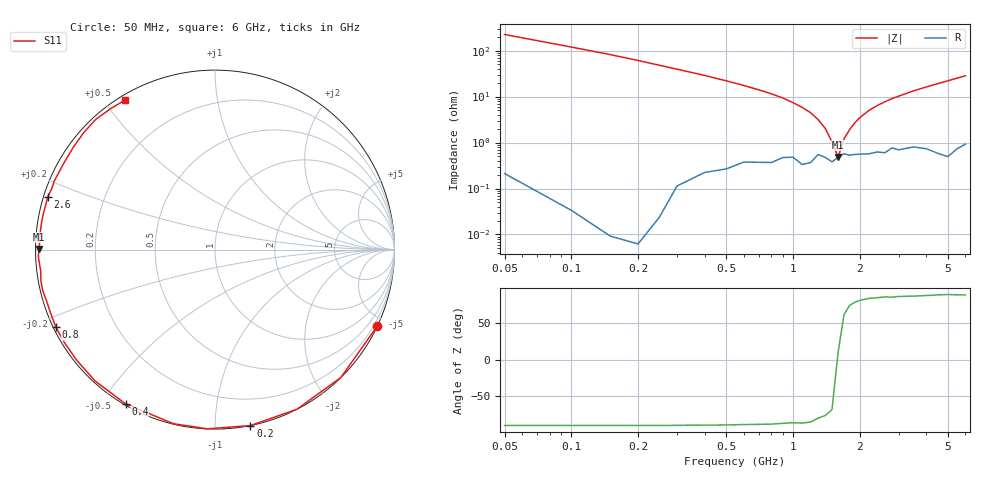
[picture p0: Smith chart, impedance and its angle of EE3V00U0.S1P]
! Infineon Technologies  Discrete & RF Semiconductors
! BBY55-02W
! Si Tuning Diode in SCD-80
! VR = 3 V
! S-Parameters:  June  2000
# GHz  S  MA  R  50
!  f  S11
! GHz  MAG  ANG
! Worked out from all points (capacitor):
!   34 points, 50 MHz to 6 GHz, reference 50 ohm
!   read as one part to ground: C = 13.3 pF near 50 MHz
!   lowest |Z| = 485 mohm at 1.6 GHz (marker M1)
!   series resonance near 1.592 GHz, so ESL is about 750 pH
!   S11 on the Smith chart (normalised r, x): 50 MHz: 0.00, -4.49; 200 MHz: 0.00, -1.22; 400 MHz: 0.00, -0.58; 800 MHz: 0.01, -0.23; 2.6 GHz: 0.01, +0.15; 6 GHz: 0.02, +0.57
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0.05  0.9996 -25.1
0.1  0.9998 -45.4
0.15  0.9999 -62.8
0.2  0.9999 -78.6
0.25  0.9995 -92.4
0.3  0.9972 -103.4
0.4  0.9933 -120.1
0.5  0.9911 -132.4
0.6  0.9867 -141.5
0.7  0.9863 -148.6
0.8  0.9861 -154.1
1  0.9814 -163.2
1.1  0.9869 -166.7
1.2  0.9856 -169.8
1.3  0.9783 -172.9
1.5  0.9849 -177.8
1.6  0.9811 179.8
1.7  0.9774 177.6
2  0.978 172.2
2.4  0.9757 165.5
2.6  0.9768 162.5
3  0.9737 156.9
3.5  0.9704 150.2
4  0.9738 144.1
4.5  0.9798 138.2
5  0.9836 132.4
5.5  0.977 126.5
6  0.9724 120.9
